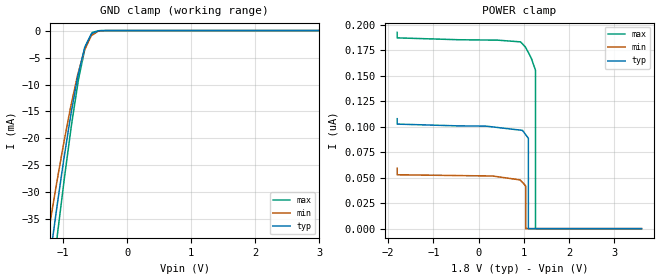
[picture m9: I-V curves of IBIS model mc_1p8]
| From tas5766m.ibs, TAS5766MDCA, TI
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|   mc_1p8 Model
[Model]   mc_1p8
Model_type   Input
Vinl = 0.54
Vinh = 1.26
|   typ   min   max
C_comp   1.056pF   1.043pF   1.074pF
[Voltage Range]   1.8   1.65   1.95
[Temperature Range]   27   105   -25
[Power Clamp Reference]   1.8   1.65   1.95
[GND Clamp Reference]   -0   -0   -0
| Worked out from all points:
|   GND clamp passes 1 mA (typ) near -0.57 V on its own axis
[GND Clamp]
|   Voltage   I(typ)   I(min)   I(max)
-1.8V     -98.84mA   -82.48mA   -114.6mA
-1.298V   -50.51mA   -42.59mA   -59.31mA
-1.207V   -42.37mA   -35.9mA    -49.89mA
-1.19V    -40.81mA   -34.64mA   -48.04mA
-1.099V   -32.99mA   -28.23mA   -38.95mA
-1.082V   -31.51mA   -27.03mA   -37.16mA
-878.7mV  -15.59mA   -14.01mA   -18.41mA
-757.7mV  -7.859mA   -7.596mA   -8.948mA
-649.7mV  -2.844mA   -3.242mA   -2.862mA
-541.7mV  -476.5uA   -815.2uA   -330uA
-343.5mV  -2.947uA   -9.62uA    -2.339uA
3.6V      0A         0A         0A
[POWER Clamp]
|   Voltage   I(typ)   I(min)   I(max)
-1.8V     107.8nA    59.16nA    192.3nA
925.6mV   96.53nA    47.38nA    183.1nA
1.042V    92.01nA    41.31nA    177.3nA
1.042V    91.98nA    0A         177.3nA
1.099V    88.45nA    0A         172.5nA
1.099V    81.67nA    0A         172.5nA
1.099V    0A         0A         172.5nA
1.257V    0A         0A         155.1nA
1.257V    0A         0A         139.7nA
1.257V    0A         0A         91.4nA
1.257V    0A         0A         0A
3.6V      0A         0A         0A
